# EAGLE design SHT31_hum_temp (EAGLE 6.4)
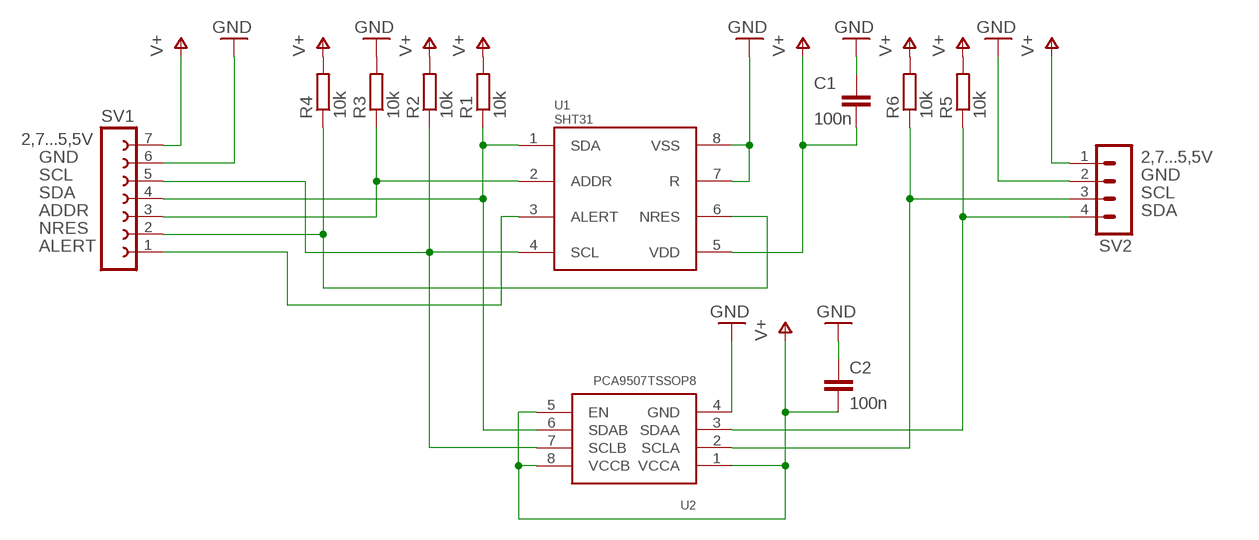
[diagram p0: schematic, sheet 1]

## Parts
C1  100n  C-EUC0805  [C0805]
C2  100n  C-EUC0805  [C0805]
R1  10k  R-EU_M0805  [M0805]
R2  10k  R-EU_M0805  [M0805]
R3  10k  R-EU_M0805  [M0805]
R4  10k  R-EU_M0805  [M0805]
R5  10k  R-EU_M0805  [M0805]
R6  10k  R-EU_M0805  [M0805]
SV1  FE07-1  [FE07]
SV2  MA04-1  [MA04-1]
U1  SHT31  SHT3X  [SHT3X]
U2  PCA9507TSSOP8  [TSSOP8]

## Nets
GND: C1.1 C2.1 R3.2 SV1.6 SV2.2 U1.7(R) U1.8(VSS) U2.4(GND)
N$1: R1.1 SV1.4 U1.1(SDA) U2.6(SDAB)
N$2: R2.1 SV1.5 U1.4(SCL) U2.7(SCLB)
N$3: R3.1 SV1.3 U1.2(ADDR)
N$4: R4.1 SV1.2 U1.6(NRES)
N$7: R6.1 SV2.3 U2.2(SCLA)
N$8: R5.1 SV2.4 U2.3(SDAA)
N$9: SV1.1 U1.3(ALERT)
V+: C1.2 C2.2 R1.2 R2.2 R4.2 R5.2 R6.2 SV1.7 SV2.1 U1.5(VDD) U2.1(VCCA) U2.5(EN) U2.8(VCCB)

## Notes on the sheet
- 2,7...5,5V
- GND | 2,7...5,5V
- SCL | GND
- SDA | SCL
- ADDR | SDA
- NRES
- ALERT

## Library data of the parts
C1 C2 = moja_biblioteka:C-EU: CAPACITOR, European symbol; SPICEPREFIX: C
R1-R6 = moja_biblioteka:R-EU_: RESISTOR, European symbol; SPICEPREFIX: R
SV1 = con-lsta:FE07-1: FEMALE HEADER; OC_FARNELL: unknown; OC_NEWARK: unknown
SV2 = con-lstb:MA04-1: PIN HEADER; OC_FARNELL: unknown; OC_NEWARK: unknown
U1 = moja_biblioteka:SHT3X: SHT3x czujnik temperatury i wilgotności SENSIRION
U2 = moja_biblioteka:PCA9507: PCA9507 2 przewodowy ekstender 2,5 - 5,5V

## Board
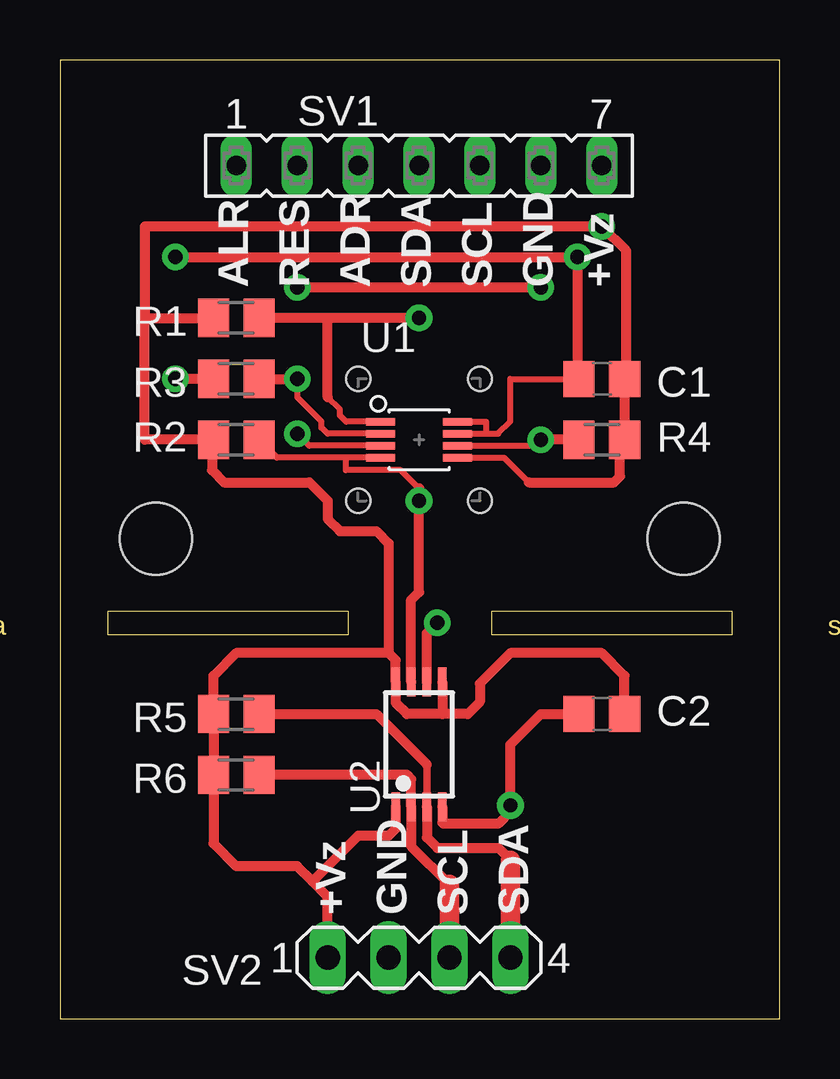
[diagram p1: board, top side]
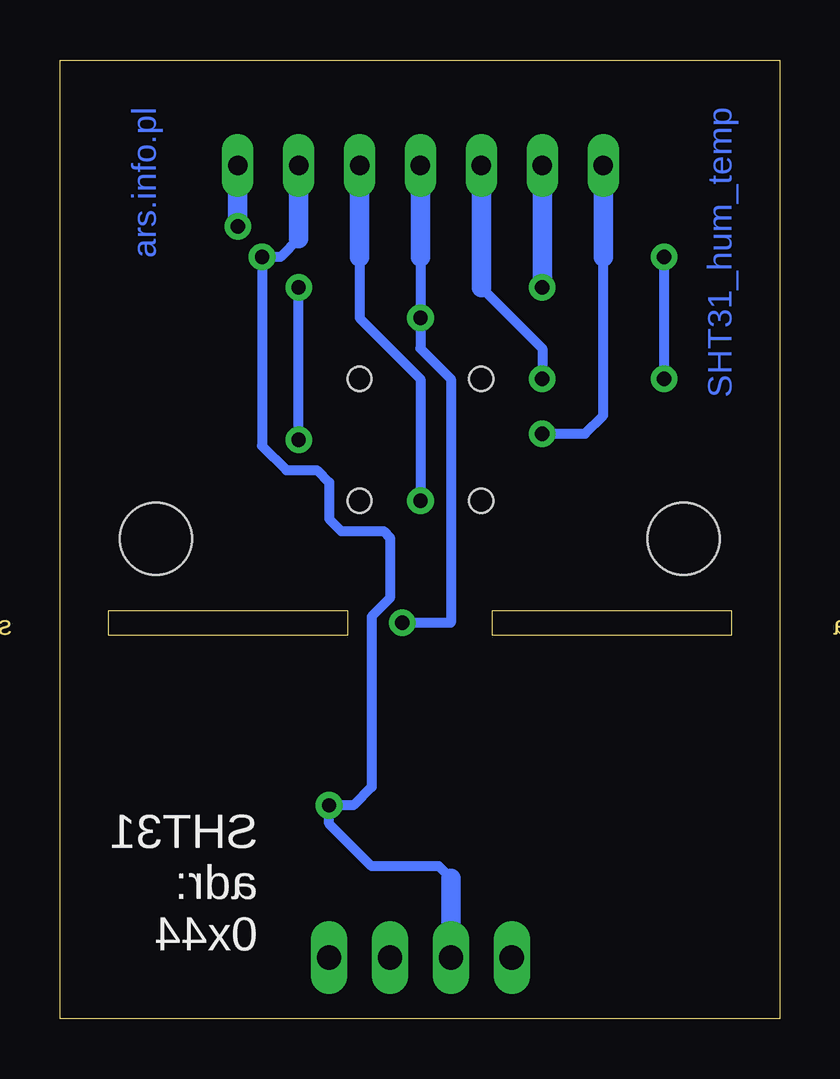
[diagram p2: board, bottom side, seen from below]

Size 30 x 39.96 mm. Coordinates in mm from the lower left corner, seen from the top.
Outline: 0,0 30,0 30,39.96 0,39.96 0,0
Outline: 2,17 12,17 12,16 2,16 2,17
Outline: 18,17 28,17 28,16 18,16 18,17
Copper layers (1*16): Top 0.035mm / dielectric 1.5mm / Bottom 0.035mm
Design rules "AVT *": minimum track width 10mil, minimum drill 19mil, track to track 7mil, track to pad 7mil, pad to pad 7mil, via to via 7mil, smd to smd 7mil, copper to edge 20mil, drill to drill 10mil, minimum pad ring 10mil, minimum via ring 10mil, stop-mask expansion 4mil, vias tented up to drill 0mil, thermal gap 10mil
Holes 1 mm at 12.43,26.67 17.51,26.67 17.51,21.59 12.43,21.59
Holes 3 mm at 4,20 26,20

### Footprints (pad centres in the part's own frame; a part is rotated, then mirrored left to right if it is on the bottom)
C0805 = smd 1.3 x 1.5: 1 -0.95,0; 2 0.95,0
M0805 = smd 1.3 x 1.6: 1 -0.95,0; 2 0.95,0
FE07 = drill 0.813 long: 1 -7.62,0; 2 -5.08,0; 3 -2.54,0; 4 0,0; 5 2.54,0; 6 5.08,0; 7 7.62,0
MA04-1 = drill 1.016 long: 1 -3.81,0; 2 -1.27,0; 3 1.27,0; 4 3.81,0
SHT3X = smd 1.2 x 0.3: 1 -1.6,0.75; 2 -1.6,0.25; 3 -1.6,-0.25; 4 -1.6,-0.75; 5 1.6,-0.75; 6 1.6,-0.25; 7 1.6,0.25; 8 1.6,0.75
TSSOP8 = smd 0.35 x 1.2: 1 -0.975,-2.6; 2 -0.325,-2.6; 3 0.325,-2.6; 4 0.975,-2.6; 5 0.975,2.6; 6 0.325,2.6; 7 -0.325,2.6; 8 -0.975,2.6

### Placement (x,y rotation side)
C1  22.59,26.67 0 top
C2  22.59,12.7 0 top
R1  7.35,29.21 180 top
R2  7.35,24.13 180 top
R3  7.35,26.67 180 top
R4  22.59,24.13 0 top
R5  7.35,12.7 180 top
R6  7.35,10.16 180 top
SV1  14.97,35.56 0 top
SV2  14.97,2.54 0 top
U1  14.97,24.13 0 top
U2  14.97,11.43 0 top

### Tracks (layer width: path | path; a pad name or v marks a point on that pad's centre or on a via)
GND  (via drill 0.6)
  Top 0.254: U1.7 17.76,24.38 | 17.76,24.38 18.27,24.38 18.78,24.89 18.78,26.67 C1.1 | U1.8 17.76,24.88 17.76,24.38
  Top 0.406: C1.1 21.57,26.74 v21.57,31.75 v4.81,31.75 | R3.2 v4.81,26.67 | U2.4 15.95,8.17 15.99,8.13 18.27,8.13 18.78,8.64 v18.78,8.89 18.78,11.43 20.05,12.7 C2.1
  Bottom 0.406: 20.05,32.51 20.81,31.75 v21.57,31.75 21.57,23.88 20.56,22.86 19.29,22.86 18.78,22.35 18.78,20.83 18.27,20.32 16.49,20.32 16.24,20.07 16.24,17.53 17,16.76 17,9.65 17.76,8.89 v18.78,8.89 18.78,8.13 17,6.35 14.21,6.35 13.7,5.84 | v4.81,26.67 v4.81,31.75
  Bottom 0.813: SV1.6 20.05,32.51 | SV2.2 13.7,5.84
N$1  (via drill 0.6)
  Top 0.254: U1.1 11.93,24.88 11.67,25.15 11.67,25.4 11.16,25.91
  Top 0.406: 11.16,25.91 11.16,29.21 | 11.16,29.21 R1.1 | v14.97,29.21 11.16,29.21 | U2.6 15.29,16.07 v15.73,16.51
  Bottom 0.406: 14.97,31.75 v14.97,29.21 14.97,27.94 13.7,26.67 13.7,16.51 v15.73,16.51
  Bottom 0.813: SV1.4 14.97,31.75
N$2  (via drill 0.6)
  Top 0.254: U1.4 11.92,23.38 | 11.92,23.38 9.05,23.38 R2.1 | 14.97,22.1 14.21,22.86 11.92,22.86 11.92,23.38
  Top 0.406: 14.97,22.1 v14.97,21.59 14.97,17.78 14.64,17.45 U2.7
  Bottom 0.406: 17.51,31.75 17.51,29.21 14.97,26.67 v14.97,21.59
  Bottom 0.813: SV1.5 17.51,31.75
N$3  (via drill 0.6)
  Top 0.254: U1.2 11.16,24.38 10.91,24.64 10.91,24.89 9.89,25.91 v9.89,26.67
  Top 0.406: R3.1 v9.89,26.67
  Bottom 0.406: 12.43,30.48 9.89,27.94 v9.89,26.67
  Bottom 0.813: SV1.3 12.43,30.48
N$4  (via drill 0.6)
  Top 0.254: U1.6 19.8,23.88 v20.05,24.13
  Top 0.406: v20.05,30.48 v9.89,30.48 | R4.1 v20.05,24.13
  Bottom 0.406: v20.05,24.13 v20.05,30.48
  Bottom 0.813: v9.89,30.48 SV1.2
N$7
  Top 0.406: 16.24,5.59 14.64,7.18 U2.2 14.64,9.98 14.46,10.16 R6.1
  Top 0.813: 16.24,5.59 SV2.3
N$8
  Top 0.305: U2.3 15.29,10.6
  Top 0.406: R5.1 13.19,12.7 15.29,10.6 | U2.3 15.29,7.55 15.73,7.11 18.27,7.11 18.78,6.6
  Top 0.813: 18.78,6.6 SV2.4
N$9  (via drill 0.6)
  Top 0.254: U1.3 10.39,23.88 v9.89,24.38
  Bottom 0.406: v9.89,24.38 8.11,24.38 7.35,25.15 7.35,31.75
  Bottom 0.813: 7.35,31.75 SV1.1
V+  (via drill 0.6)
  Top 0.254: U1.5 18.51,23.38 19.54,22.35 | 23.35,23.94 R4.2 23.86,24.13
  Top 0.406: R2.2 6.33,24.13 | 6.33,24.13 3.54,24.13 3.54,29.21 | 3.54,29.21 R1.2 | 19.54,22.35 23.1,22.35 23.35,22.61 23.35,23.94 | R4.2 C1.2 23.61,26.67 23.61,32 v22.59,33.02 3.54,33.02 3.54,29.21 | SV2.1 11.16,5.08 10.53,5.71 | 10.53,5.71 9.89,6.35 7.35,6.35 6.4,7.3 R6.2 R5.2 6.4,14.29 7.35,15.24 13.7,15.24 | U2.1 13.99,7.92 13.7,7.62 12.43,7.62 10.53,5.71 | 13.7,15.24 13.99,14.95 U2.8 13.99,13.17 14.46,12.7 15.95,12.7 | U2.5 15.95,12.7 | C2.2 23.54,14.29 22.59,15.24 18.78,15.24 17.51,13.97 17.51,13.21 17,12.7 15.95,12.7 | 6.33,24.13 6.33,22.86 6.84,22.35 10.4,22.35 11.16,21.59 11.16,20.83 11.67,20.32 13.19,20.32 13.7,19.81 13.7,15.24
  Bottom 0.813: v22.59,33.02 SV1.7

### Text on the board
Bottom: SHT31_hum_temp | ars.info.pl
Dimension: szczelina | szczelina
tNames: ALR | RES | ADR | SDA | SCL | GND | +Vz | +Vz | GND | SCL | SDA
bNames: SHT31 / adr: / 0x44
